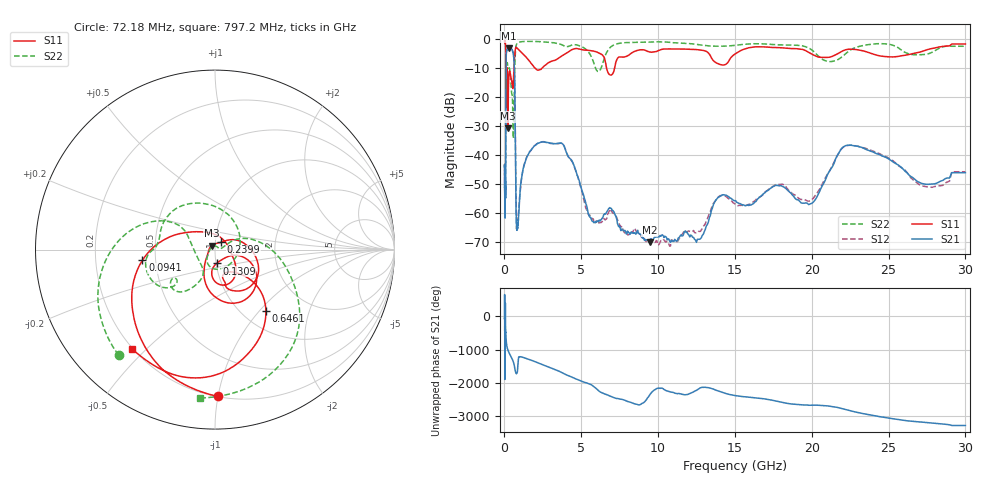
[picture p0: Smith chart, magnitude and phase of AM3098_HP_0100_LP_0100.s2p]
! Date/Time: Thu, Feb 28, 2019 8:35 AM
! Network Analyzer: Agilent Technologies E8364B Rev: A.07.50.67
! Sweep from 0.010 to 30.000 GHz, 1601 Points, Sweep Type: LOG
! Power Supply: 5.022 V, 0.002 A
# Hz S DB R 50
!freq MagS11 AngS11 MagS21 AngS21 MagS12 AngS12 MagS22 AngS22
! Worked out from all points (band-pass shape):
!   1601 points, 10 MHz to 30 GHz, reference 50 ohm
!   highest |S21| = -3.03 dB at 266.5 MHz (marker M1); lowest = -70.2 dB at 9.443 GHz (marker M2)
!   |S21| within 3 dB of the highest: 111.1 MHz to 601.6 MHz (490.5 MHz wide, 138 % of centre)
!   lowest |S11| = -30.7 dB at 229.3 MHz (marker M3), VSWR 1.06, Z = 48.1 + j2.09 ohm
!   |S11| at or under -10 dB: 177.1 MHz to 619.2 MHz (442.1 MHz wide, 111 % of centre); 2.013 GHz to 2.428 GHz (415.1 MHz wide, 18.7 % of centre); 6.649 GHz to 7.164 GHz (515 MHz wide, 7.46 % of centre)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
!   |S22| runs from -34.2 to -0.5 dB; largest |S21 - S12| = 0.011
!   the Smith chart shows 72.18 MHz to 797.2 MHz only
!   S11 on the Smith chart (normalised r, x): 72.18 MHz: 0.20, -1.00; 94.1 MHz: 0.42, -0.06; 130.9 MHz: 1.00, -0.16; 239.9 MHz: 1.07, +0.09; 646.1 MHz: 1.28, -1.08; 797.2 MHz: 0.20, -0.45
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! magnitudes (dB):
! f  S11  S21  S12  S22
! 10 MHz  -0.3  -44.2  -43.3  -0.5
! 38.04 MHz  -0.5  -58.4  -58.8  -0.8
! 72.18 MHz  -1.8  -54.5  -54.4  -2.0
! 94.1 MHz  -7.8  -20.8  -20.8  -9.4
! 103.5 MHz  -22.7  -8.5  -8.5  -17.9
! 130.9 MHz  -22.2  -4.2  -4.2  -11.0
! 144.7 MHz  -15.7  -3.7  -3.7  -10.7
! 185.8 MHz  -11.0  -3.5  -3.5  -8.1
! 229.3 MHz  -30.7  -3.1  -3.1  -9.6
! 239.9 MHz  -25.5  -3.1  -3.1  -9.8
! 266.5 MHz  -15.1  -3.0  -3.0  -10.0
! 550.5 MHz  -16.8  -4.4  -4.3  -30.2
! 646.1 MHz  -7.1  -10.2  -10.2  -15.3
! 797.2 MHz  -2.8  -65.3  -65.1  -1.6
! 2.084 GHz  -10.4  -36.2  -36.1  -0.7
! 3.798 GHz  -5.5  -36.2  -36.1  -2.0
! 5.668 GHz  -3.9  -62.4  -61.6  -6.1
! 7.926 GHz  -5.9  -67.2  -66.9  -1.1
! 9.443 GHz  -4.3  -70.2  -70.0  -0.9
! 19.7 GHz  -4.2  -56.6  -55.8  -2.7
! 22.67 GHz  -3.4  -36.7  -36.6  -3.2
! 30 GHz  -1.6  -46.1  -45.7  -2.3
